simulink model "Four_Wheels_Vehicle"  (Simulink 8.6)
settings: Solver=ode45  StartTime=0.0  StopTime=20  RelTol=1e-3
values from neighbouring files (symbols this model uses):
  beta = 1    [Vehicle_Parameters.m]
  g = 9.81    [Vehicle_Parameters.m]
  H_CoG = 0.700    (= 0.7)    [Vehicle_Parameters.m]
  Hearo = 0.750    (= 0.75)    [Vehicle_Parameters.m]
  Iz = 2480    [Vehicle_Parameters.m]
  Jw = 2.166    [Vehicle_Parameters.m]
  L = 10    [Vehicle_Parameters.m]
  Lf = 1.180    (= 1.18)    [Vehicle_Parameters.m]
  Lr = 1.770    (= 1.77)    [Vehicle_Parameters.m]
  Lw = 1.880    (= 1.88)    [Vehicle_Parameters.m]
  m = 1500    [Vehicle_Parameters.m]
  miu = 0.85    [Vehicle_Parameters.m]
  reff = 0.380    (= 0.38)    [Vehicle_Parameters.m]
undefined symbols (not defined in the file or in its folder): DiscIntNeverNeededParam, Init, Ki, Kp, LowerLimit, sigbuilder_block, Ts, UpperLimit
libraries: simulink x15, powerlib_extras x3
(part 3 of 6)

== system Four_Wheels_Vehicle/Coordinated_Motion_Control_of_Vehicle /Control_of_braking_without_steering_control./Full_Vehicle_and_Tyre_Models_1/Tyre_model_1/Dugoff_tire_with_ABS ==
  note: Dugoff_Tire_model
  In1 : Inport
  In2 : Inport  Port=2
  In5 : Inport  Port=3
  In3 : Inport  Port=4
  Demux{1..4} (4 alike) : Demux  Outputs=3
  Dugoff_Tire_FL : MATLAB Function  TreatAsAtomicUnit=on
  Dugoff_Tire_FR : MATLAB Function  TreatAsAtomicUnit=on
  Dugoff_Tire_RL : MATLAB Function  TreatAsAtomicUnit=on
  Dugoff_Tire_RR : MATLAB Function  TreatAsAtomicUnit=on
  miu{,1..3} (4 alike) : Constant  Value=miu
  Fx_FL_1 : Outport
  Fx_FR_1 : Outport  Port=2
  Fy_FL_1 : Outport  Port=3
  Fy_FR_1 : Outport  Port=4
  Fx_RL_1 : Outport  Port=5
  Fx_RR_1 : Outport  Port=6
  Fy_RL_1 : Outport  Port=7
  Fy_RR_1 : Outport  Port=8
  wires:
  In3/1 -> Demux3/1
  Demux1/3 -> Dugoff_Tire_RR/3(alpha_RR)
  Demux1/1 -> Dugoff_Tire_RR/1(Sigma)
  Demux3/1 -> Dugoff_Tire_RL/1(Sigma)
  Demux3/3 -> Dugoff_Tire_RL/3(alpha_RL)
  In2/1 -> Demux2/1
  Dugoff_Tire_RR/2(Fy_RR) -> Fy_RR_1/1
  Dugoff_Tire_RL/2(Fy_RL) -> Fy_RL_1/1
  Dugoff_Tire_RR/1(Fx_RR) -> Fx_RR_1/1
  Dugoff_Tire_RL/1(Fx_RL) -> Fx_RL_1/1
  In5/1 -> Demux1/1
  Dugoff_Tire_FR/2(Fy_FR) -> Fy_FR_1/1
  Dugoff_Tire_FL/2(Fy_FL) -> Fy_FL_1/1
  Dugoff_Tire_FR/1(Fx_FR) -> Fx_FR_1/1
  Dugoff_Tire_FL/1(Fx_FL) -> Fx_FL_1/1
  In1/1 -> Demux4/1
  miu3/1 -> Dugoff_Tire_RR/4(miu)
  miu2/1 -> Dugoff_Tire_RL/4(miu)
  miu/1 -> Dugoff_Tire_FR/4(miu)
  miu1/1 -> Dugoff_Tire_FL/4(miu)
  Demux4/1 -> Dugoff_Tire_FL/1(Sigma)
  Demux4/2 -> Dugoff_Tire_FL/2(Fz_FL)
  Demux4/3 -> Dugoff_Tire_FL/3(alpha_FL)
  Demux3/2 -> Dugoff_Tire_RL/2(Fz_RL)
  Demux2/1 -> Dugoff_Tire_FR/1(Sigma)
  Demux2/2 -> Dugoff_Tire_FR/2(Fz_FR)
  Demux2/3 -> Dugoff_Tire_FR/3(alpha_FR)
  Demux1/2 -> Dugoff_Tire_RR/2(Fz_RR)

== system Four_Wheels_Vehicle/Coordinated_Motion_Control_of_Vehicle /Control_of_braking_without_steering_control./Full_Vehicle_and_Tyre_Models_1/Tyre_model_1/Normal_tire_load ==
  x_Vel_1 : Inport
  mass : Inport  Port=2
  g : Inport  Port=3
  H_CoG : Inport  Port=4
  beta : Inport  Port=5
  Lf : Inport  Port=6
  Lr : Inport  Port=7
  Hearo : Inport  Port=8
  AirDragConst : Constant  Value=0.3
  Airdensity : Constant  Value=1.22
  Constant : Constant  Value=2
  Constant1 : Constant  Value=2
  Divide : Product  Inputs=*/
  Divide1 : Product  Inputs=*/
  Faero : Subsystem
  FrontalArea : Constant  Value=2
  Fzf : Subsystem
  Fzr : Subsystem
  Scope : Scope
  windVelocity : Constant
  Fz_f_1 : Outport
  Fz_r_1 : Outport  Port=2
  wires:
  Faero/1(Faero) -> Scope/1, Fzf/9(Faero), Fzr/1(Faero)
  x_Vel_1/1 -> Fzr/3(xVel), Fzf/1(x_Vel), Faero/1(Vx)
  windVelocity/1 -> Faero/5(windVelocity)
  Airdensity/1 -> Faero/4(Airdensity)
  FrontalArea/1 -> Faero/3(FrontalArea1)
  AirDragConst/1 -> Faero/2(AirDragConst1)
  mass/1 -> Fzr/4(mass), Fzf/2(mass)
  Hearo/1 -> Fzr/2(Haero), Fzf/8(Haero)
  H_CoG/1 -> Fzr/6(HatCG), Fzf/4(H_CoG)
  g/1 -> Fzr/5(g), Fzf/3(g)
  Divide1/1 -> Fz_r_1/1
  Divide/1 -> Fz_f_1/1
  Constant1/1 -> Divide1/2
  Constant/1 -> Divide/2
  Fzr/1(Fzr) -> Divide1/1
  Fzf/1(Fz_f) -> Divide/1
  Lf/1 -> Fzr/8(Lf), Fzf/6(Lf)
  beta/1 -> Fzr/7(beta), Fzf/5(beta)
  Lr/1 -> Fzr/9(Lr), Fzf/7(Lr)

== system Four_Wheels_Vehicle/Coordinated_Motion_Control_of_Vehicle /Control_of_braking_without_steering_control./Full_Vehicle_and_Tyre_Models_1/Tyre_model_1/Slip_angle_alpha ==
  note: Slip_angle_alpha
  x_Vel_1 : Inport
  y_Vel_1 : Inport  Port=2
  yaw_rate_1 : Inport  Port=3
  Steering_Ang._1 : Inport  Port=4
  Lf : Constant  Value=Lf
  Lr : Constant  Value=Lr
  Slip_angle_alpha : MATLAB Function  TreatAsAtomicUnit=on
  alpha_FL_1 : Outport
  alpha_FR_1 : Outport  Port=2
  alpha_RL_1 : Outport  Port=3
  alpha_RR_1 : Outport  Port=4
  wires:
  Steering_Ang._1/1 -> Slip_angle_alpha/6(deltaw)
  Lr/1 -> Slip_angle_alpha/5(Lr)
  Lf/1 -> Slip_angle_alpha/4(Lf)
  yaw_rate_1/1 -> Slip_angle_alpha/3(yaw_rate)
  y_Vel_1/1 -> Slip_angle_alpha/2(y_Vel)
  x_Vel_1/1 -> Slip_angle_alpha/1(x_Vel)
  Slip_angle_alpha/1(alpha_FL) -> alpha_FL_1/1
  Slip_angle_alpha/2(alpha_FR) -> alpha_FR_1/1
  Slip_angle_alpha/3(alpha_RL) -> alpha_RL_1/1
  Slip_angle_alpha/4(alpha_RR) -> alpha_RR_1/1

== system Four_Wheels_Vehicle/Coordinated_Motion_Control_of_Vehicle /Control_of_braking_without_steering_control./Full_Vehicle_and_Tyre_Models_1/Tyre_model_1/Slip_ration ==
  note: Slip_ration
  Omega_FL_1 : Inport
  Omega_FR_1 : Inport  Port=2
  Omega_RL_1 : Inport  Port=3
  Omega_RR_1 : Inport  Port=4
  x_Vel_1 : Inport  Port=5
  Slip_ration_Sigma : MATLAB Function  TreatAsAtomicUnit=on
  reff : Constant  Value=reff
  Sigma_FL_1 : Outport
  Sigma_FR_1 : Outport  Port=2
  Sigma_RL_1 : Outport  Port=3
  Sigma_RR_1 : Outport  Port=4
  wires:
  x_Vel_1/1 -> Slip_ration_Sigma/5(x_Vel)
  Omega_FR_1/1 -> Slip_ration_Sigma/2(Omega_FR)
  Omega_RR_1/1 -> Slip_ration_Sigma/4(Omega_RR)
  Omega_RL_1/1 -> Slip_ration_Sigma/3(Omega_RL)
  Omega_FL_1/1 -> Slip_ration_Sigma/1(Omega_FL)
  Slip_ration_Sigma/1(Sigma_FL) -> Sigma_FL_1/1
  Slip_ration_Sigma/4(Sigma_RR) -> Sigma_RR_1/1
  Slip_ration_Sigma/3(Sigma_RL) -> Sigma_RL_1/1
  Slip_ration_Sigma/2(Sigma_FR) -> Sigma_FR_1/1
  reff/1 -> Slip_ration_Sigma/6(reff)

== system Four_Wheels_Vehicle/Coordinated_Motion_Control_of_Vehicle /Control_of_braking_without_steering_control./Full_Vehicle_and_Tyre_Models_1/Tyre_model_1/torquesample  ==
  Demux : Demux  Tag=STV Demux  Outputs=1
  FromWs : FromWorkspace  Tag=STV FromWs  VariableName=tuvar  SampleTime=0  SigBuilderData=DataTag4  VnvData=DataTag5
  Signal 1 : Outport  Tag=STV Outport
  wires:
  Demux/1 -> Signal 1/1
  FromWs/1 -> Demux/1

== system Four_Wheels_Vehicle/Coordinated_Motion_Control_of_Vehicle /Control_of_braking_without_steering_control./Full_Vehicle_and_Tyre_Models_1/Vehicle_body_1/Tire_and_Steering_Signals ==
  Steering_Ang. : Inport
  Fx_and_Fy : Inport  Port=2
  Demux : Demux  Outputs=8
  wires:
  Fx_and_Fy/1 -> Demux/1
  Demux/8 -> [Fy_RR_1]
  Demux/7 -> [Fy_RL_1]
  Demux/6 -> [Fx_RR_1]
  Demux/5 -> [Fx_RL_1]
  Demux/4 -> [Fy_FR_1]
  Demux/3 -> [Fy_FL_1]
  Demux/2 -> [Fx_FR_1]
  Demux/1 -> [Fx_FL_1]
  Steering_Ang./1 -> [SteeringAng_1]

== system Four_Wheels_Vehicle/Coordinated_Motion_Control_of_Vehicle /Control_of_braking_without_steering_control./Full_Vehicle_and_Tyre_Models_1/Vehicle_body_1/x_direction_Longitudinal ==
  note: x_direction_Longitudinal
  Fx_FL_1 : Inport
  Fx_FR_1 : Inport  Port=2
  Fy_FL_1 : Inport  Port=3
  Fy_FR_1 : Inport  Port=4
  Fx_RL_1 : Inport  Port=5
  Fx_RR_1 : Inport  Port=6
  Steering_Ang_1 : Inport  Port=7
  yaw_rate_1 : Inport  Port=8
  y_Vel_1 : Inport  Port=9
  1/m : Gain  Gain=1/1750
  Add : Sum
  Add1 : Sum
  Add2 : Sum  Inputs=+-++
  Add3 : Sum
  Product : Product
  Product1 : Product
  Product18 : Product
  Stop Simulation : Stop
  Vx0 : Integrator  InitialCondition=5  UpperSaturationLimit=100  LowerSaturationLimit=0  ShowSaturationPort=on
  cos_deltaw : Fcn  Expr=cos(u)
  sin_deltaw : Fcn  Expr=sin(u)
  x_Vel_1 : Outport
  x total force : Outport  Port=2
  dx : Outport  Port=3
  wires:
  Fx_RR_1/1 -> Add2/4
  Fx_RL_1/1 -> Add2/3
  Product1/1 -> Add2/2
  Product/1 -> Add2/1
  Fx_FR_1/1 -> Add/2
  Fx_FL_1/1 -> Add/1
  Fy_FR_1/1 -> Add1/2
  Fy_FL_1/1 -> Add1/1
  sin_deltaw/1 -> Product1/2
  Add1/1 -> Product1/1
  y_Vel_1/1 -> Product18/2
  yaw_rate_1/1 -> Product18/1
  Steering_Ang_1/1 -> sin_deltaw/1, cos_deltaw/1
  Add/1 -> Product/1
  cos_deltaw/1 -> Product/2
  Add2/1 -> x total force/1, 1/m/1
  1/m/1 -> Add3/1
  Add3/1 -> Vx0/1, dx/1
  Vx0/2 -> Stop Simulation/1
  Vx0/1 -> x_Vel_1/1
  Product18/1 -> Add3/2

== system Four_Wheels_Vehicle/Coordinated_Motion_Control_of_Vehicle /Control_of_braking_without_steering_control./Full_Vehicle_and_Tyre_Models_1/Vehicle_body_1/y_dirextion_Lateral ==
  note: y_dirextion_Lateral
  Fx_FL_1 : Inport
  Fx_FR_1 : Inport  Port=2
  Fy_FL_1 : Inport  Port=3
  Fy_FR_1 : Inport  Port=4
  Fy_RL_1 : Inport  Port=5
  Fy_RR_1 : Inport  Port=6
  Steering_Ang._1 : Inport  Port=7
  yaw_rate_1 : Inport  Port=8
  x_Vel_1 : Inport  Port=9
  1/m : Gain  Gain=1/1750
  Add1 : Sum
  Add12 : Sum
  Add15 : Sum  Inputs=++++
  Add2 : Sum  Inputs=+-
  Product1 : Product
  Product13 : Product
  Product3 : Product
  Vx0 : Integrator  UpperSaturationLimit=50/3.6  LowerSaturationLimit=eps
  cos_deltaw2 : Fcn  Expr=cos(u)
  sin_deltaw2 : Fcn  Expr=sin(u)
  y_Vel_1 : Outport
  y total force : Outport  Port=2
  dy : Outport  Port=3
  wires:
  Add2/1 -> Vx0/1, dy/1
  Fy_RL_1/1 -> Add15/3
  Fy_RR_1/1 -> Add15/4
  Product13/1 -> Add15/1
  Product1/1 -> Add15/2
  Fx_FR_1/1 -> Add12/2
  Fx_FL_1/1 -> Add12/1
  Fy_FR_1/1 -> Add1/2
  Fy_FL_1/1 -> Add1/1
  Product3/1 -> Add2/2
  x_Vel_1/1 -> Product3/2
  yaw_rate_1/1 -> Product3/1
  cos_deltaw2/1 -> Product1/2
  Add1/1 -> Product1/1
  Vx0/1 -> y_Vel_1/1
  1/m/1 -> Add2/1
  Add15/1 -> y total force/1, 1/m/1
  sin_deltaw2/1 -> Product13/2
  Add12/1 -> Product13/1
  Steering_Ang._1/1 -> cos_deltaw2/1, sin_deltaw2/1

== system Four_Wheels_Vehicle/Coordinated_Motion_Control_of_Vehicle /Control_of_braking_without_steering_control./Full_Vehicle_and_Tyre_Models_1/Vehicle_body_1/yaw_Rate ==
  note: yaw_Rate_and_z_torque
  Fx_FL_1 : Inport
  Fx_FR_1 : Inport  Port=2
  Fy_FL_1 : Inport  Port=3
  Fy_FR_1 : Inport  Port=4
  Fx_RL_1 : Inport  Port=5
  Fx_RR_1 : Inport  Port=6
  Fy_RL_1 : Inport  Port=7
  Fy_RR_1 : Inport  Port=8
  Steering_Ang._1 : Inport  Port=9
  1/Iz : Gain  Gain=1/Iz
  Add1 : Sum  Inputs=-+
  Add10 : Sum  Inputs=+++++-
  Add2 : Sum
  Add3 : Sum  Inputs=-+
  Add4 : Sum
  Add5 : Sum  Inputs=-+
  Add6 : Sum
  Integrator1 : Integrator  InitialCondition=eps  UpperSaturationLimit=50/3.6  LowerSaturationLimit=eps  ShowSaturationPort=on
  Lf : Constant  Value=Lf
  Lr : Constant  Value=Lr
  Lw/2 : Constant  Value=Lw/2
  Product{1..9,13} (10 alike) : Product
  Stop Simulation1 : Stop
  cosdeltaw1 : Fcn  Expr=cos(u)
  sindeltaw1 : Fcn  Expr=sin(u)
  yaw_rate_1 : Outport
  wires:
  Fy_RR_1/1 -> Add6/2
  Fy_RL_1/1 -> Add6/1
  Fx_RR_1/1 -> Add5/2
  Fx_RL_1/1 -> Add5/1
  Fx_FR_1/1 -> Add1/2, Add4/2
  Fx_FL_1/1 -> Add1/1, Add4/1
  Fy_FL_1/1 -> Add2/1, Add3/2
  Fy_FR_1/1 -> Add3/1, Add2/2
  Add10/1 -> 1/Iz/1
  Add3/1 -> Product6/2
  Product6/1 -> Product5/1
  Product5/1 -> Add10/4
  Product9/1 -> Add10/5
  Product8/1 -> Add10/6
  Product2/1 -> Add10/3
  Product7/1 -> Product13/2
  Product13/1 -> Add10/2
  Add6/1 -> Product8/1
  Add5/1 -> Product9/1
  Add2/1 -> Product7/1
  Product4/1 -> Product2/1
  Product1/1 -> Product3/1
  Integrator1/2 -> Stop Simulation1/1
  Integrator1/1 -> yaw_rate_1/1
  1/Iz/1 -> Integrator1/1
  Product3/1 -> Add10/1
  Lr/1 -> Product8/2
  Lw/2/1 -> Product9/2, Product2/2, Product5/2
  cosdeltaw1/1 -> Product4/2, Product7/2
  Add1/1 -> Product4/1
  Lf/1 -> Product13/1, Product3/2
  sindeltaw1/1 -> Product1/2, Product6/1
  Add4/1 -> Product1/1
  Steering_Ang._1/1 -> sindeltaw1/1, cosdeltaw1/1

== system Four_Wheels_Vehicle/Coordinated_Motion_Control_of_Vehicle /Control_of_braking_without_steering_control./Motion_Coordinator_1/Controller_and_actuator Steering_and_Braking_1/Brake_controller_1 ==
  Reference_Sideslip_1 : Inport
  Feedback_Sideslip_1 : Inport  Port=2
  Add1 : Sum
  Brake_Actuator_1 : Subsystem
  Brake_controller_1 : Subsystem
  Ramp : simulink/Sources/Ramp  slope=3  start=1  X0=0
  Sideslip_angle : Scope  NumInputPorts=2
  x_seitch2 : ManualSwitch  CurrentSetting=0
  Mzc_1 : Outport
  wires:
  x_seitch2/1 -> Add1/2
  Add1/1 -> Mzc_1/1
  Reference_Sideslip_1/1 -> Brake_controller_1/1(Reference), Sideslip_angle/1, Add1/1
  Brake_controller_1/2(Sideslip_Ang1) -> Brake_Actuator_1/1(input)
  Feedback_Sideslip_1/1 -> Brake_controller_1/2(Feedback), Sideslip_angle/2
  Ramp/1 -> x_seitch2/1
  Brake_Actuator_1/1(output) -> x_seitch2/2

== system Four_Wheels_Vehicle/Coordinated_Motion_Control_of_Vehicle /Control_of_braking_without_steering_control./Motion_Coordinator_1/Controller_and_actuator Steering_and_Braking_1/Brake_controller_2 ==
  Reference_Sideslip_2 : Inport
  Feedback_Sideslip_2 : Inport  Port=2
  Add1 : Sum
  Brake_Actuator_2 : Subsystem
  Brake_controller_2 : Subsystem
  Ramp : simulink/Sources/Ramp  slope=3  start=1  X0=0
  Sideslip_angle : Scope  NumInputPorts=2
  x_seitch2 : ManualSwitch  CurrentSetting=0
  Mzc_2 : Outport
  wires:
  Brake_Actuator_2/1(output) -> x_seitch2/2
  Ramp/1 -> x_seitch2/1
  Feedback_Sideslip_2/1 -> Sideslip_angle/2, Brake_controller_2/2(Feedback)
  Brake_controller_2/2(Sideslip_Ang1) -> Brake_Actuator_2/1(input)
  Reference_Sideslip_2/1 -> Add1/1, Sideslip_angle/1, Brake_controller_2/1(Reference)
  Add1/1 -> Mzc_2/1
  x_seitch2/1 -> Add1/2

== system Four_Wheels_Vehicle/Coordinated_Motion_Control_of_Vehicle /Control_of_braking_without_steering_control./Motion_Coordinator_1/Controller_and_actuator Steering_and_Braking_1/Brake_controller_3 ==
  Reference_Sideslip_3 : Inport
  Feedback_Sideslip_3 : Inport  Port=2
  Add1 : Sum
  Brake_Actuator_3 : Subsystem
  Brake_controller_3 : Subsystem
  Ramp : simulink/Sources/Ramp  slope=3  start=1  X0=0
  Sideslip_angle : Scope  NumInputPorts=2
  x_seitch2 : ManualSwitch  CurrentSetting=0
  Mzc_3 : Outport
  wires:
  x_seitch2/1 -> Add1/2
  Add1/1 -> Mzc_3/1
  Reference_Sideslip_3/1 -> Brake_controller_3/1(Reference), Sideslip_angle/1, Add1/1
  Brake_controller_3/2(Sideslip_Ang1) -> Brake_Actuator_3/1(input)
  Feedback_Sideslip_3/1 -> Brake_controller_3/2(Feedback), Sideslip_angle/2
  Ramp/1 -> x_seitch2/1
  Brake_Actuator_3/1(output) -> x_seitch2/2

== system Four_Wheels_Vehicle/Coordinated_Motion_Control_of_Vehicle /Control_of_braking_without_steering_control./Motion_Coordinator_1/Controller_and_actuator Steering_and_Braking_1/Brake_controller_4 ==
  Reference_Sideslip_4 : Inport
  Feedback_Sideslip_4 : Inport  Port=2
  Add1 : Sum
  Brake_Actuator_4 : Subsystem
  Brake_controller_4 : Subsystem
  Ramp : simulink/Sources/Ramp  slope=3  start=1  X0=0
  Sideslip_angle : Scope  NumInputPorts=2
  x_seitch2 : ManualSwitch  CurrentSetting=0
  Mzc_4 : Outport
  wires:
  Brake_Actuator_4/1(output) -> x_seitch2/2
  Ramp/1 -> x_seitch2/1
  Feedback_Sideslip_4/1 -> Sideslip_angle/2, Brake_controller_4/2(Feedback)
  Brake_controller_4/2(Sideslip_Ang1) -> Brake_Actuator_4/1(input)
  Reference_Sideslip_4/1 -> Add1/1, Sideslip_angle/1, Brake_controller_4/1(Reference)
  Add1/1 -> Mzc_4/1
  x_seitch2/1 -> Add1/2

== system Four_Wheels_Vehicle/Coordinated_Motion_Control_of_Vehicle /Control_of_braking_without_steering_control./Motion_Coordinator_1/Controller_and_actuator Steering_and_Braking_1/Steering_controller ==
  StteringAng : Inport
  Reference_Steering : Inport  Port=2
  Feedback_Steering : Inport  Port=3
  Add : Sum
  Steering_Actuator : Subsystem
  Steering_controller : Subsystem
  x_seitch1 : ManualSwitch
  yaw_comparsion : Scope  NumInputPorts=2
  f : Outport
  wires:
  Reference_Steering/1 -> yaw_comparsion/1, Steering_controller/1(Reference), x_seitch1/1
  StteringAng/1 -> Add/1
  x_seitch1/1 -> Add/2
  Steering_controller/2(Steering_Ang1) -> Steering_Actuator/1(input)
  Steering_Actuator/1(output) -> x_seitch1/2
  Feedback_Steering/1 -> Steering_controller/2(Feedback), yaw_comparsion/2
  Add/1 -> f/1

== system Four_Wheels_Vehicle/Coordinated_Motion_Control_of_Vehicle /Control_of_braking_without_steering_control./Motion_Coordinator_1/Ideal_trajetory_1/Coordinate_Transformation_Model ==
  note: vehicle heading
  delta_steer (rad) : Inport
  v_x (m/s) : Inport  Port=2
  1/L : Gain  Gain=1/L
  Beta : Scope
  Beta1 : Scope
  Divide : Product  Inputs=*/
  Gain : Gain  Gain=L/2
  Gain1 : Gain  Gain=0.1
  Gain2 : Gain  Gain=0.1
  Gain4 : Gain  Gain=0.345
  Ground : Ground
  Integrator : Integrator
  Integrator1 : Integrator  LimitOutput=on  UpperSaturationLimit=0
  Integrator2 : Integrator
  Product{,1,3..4} (4 alike) : Product
  Sideslip_angle : Scope
  Subtract : Sum  Inputs=+-
  Sum : Sum  Inputs=|+-
  Sum1 : Sum  Inputs=|++
  Terminator : Terminator
  Trigonometric Function : Trigonometry  Operator=cos
  Trigonometric Function1 : Trigonometry
  Trigonometric Function2 : Trigonometry  Operator=atan
  Trigonometric Function3 : Trigonometry  Operator=tan
  steerVsYawrate1 : Scope  NumInputPorts=3
  steerVsYawrate2 : Scope  NumInputPorts=3
  yaw_rate : Product
  X-position : Outport
  Y-position : Outport  Port=2
  yaw_Rate : Outport  Port=3
  Sideslip_beta : Outport  Port=4
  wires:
  Product/1 -> Sum1/1
  Product1/1 -> Sum/1
  Trigonometric Function/1 -> Product1/2, Product4/2  "cos(psi)"
  Trigonometric Function1/1 -> Product/2, Product3/2  "sin(psi)"
  Integrator2/1 -> Gain1/1  "yaw_heading (rad)"
  Integrator/1 -> steerVsYawrate1/1, X-position/1
  Integrator1/1 -> steerVsYawrate1/2, Y-position/1
  v_x (m/s)/1 -> Product/1, Product1/1, 1/L/1  "v_x (m/s)"
  yaw_rate/1 -> steerVsYawrate2/1, Gain/1, Beta1/1, Subtract/2, yaw_Rate/1, Gain2/1
  1/L/1 -> yaw_rate/1  "v_x / L"
  Sum/1 -> steerVsYawrate2/2, Integrator/1, Divide/2  "v_X (m/s)"
  Sum1/1 -> Gain4/1  "v_Y (m/s)"
  Gain/1 -> Product3/1, Product4/1  "L/2*psi-dot"
  Product3/1 -> Sum/2
  Product4/1 -> Sum1/2
  Ground/1 -> Trigonometric Function3/1
  Trigonometric Function3/1 -> Terminator/1
  Divide/1 -> Trigonometric Function2/1
  delta_steer (rad)/1 -> yaw_rate/2
  Gain1/1 -> Trigonometric Function/1, steerVsYawrate1/3, Trigonometric Function1/1
  Gain2/1 -> Integrator2/1
  Trigonometric Function2/1 -> Sideslip_angle/1, Sideslip_beta/1, Subtract/1
  Gain4/1 -> steerVsYawrate2/3, Integrator1/1, Divide/1
  Subtract/1 -> Beta/1

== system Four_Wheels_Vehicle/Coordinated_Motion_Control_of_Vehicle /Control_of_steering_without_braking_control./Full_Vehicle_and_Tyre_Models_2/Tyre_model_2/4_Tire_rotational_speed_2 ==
  Tb_FL_2 : Inport
  Tb_FR_2 : Inport  Port=2
  Tb_RL_2 : Inport  Port=3
  Tb_RR_2 : Inport  Port=4
  Td_FL_2 : Inport  Port=5
  Td_FR_2 : Inport  Port=6
  Td_RL_2 : Inport  Port=7
  Td_RR_2 : Inport  Port=8
  Fx_FL_2 : Inport  Port=9
  Fx_FR_2 : Inport  Port=10
  Fx_RL_2 : Inport  Port=11
  Fx_RR_2 : Inport  Port=12
  Tire_speed_FL : Subsystem
  Tire_speed_FR : Subsystem
  Tire_speed_RL : Subsystem
  Tire_speed_RR : Subsystem
  Omega_FL_2 : Outport
  Omega_FR_2 : Outport  Port=2
  Omega_RL_2 : Outport  Port=3
  Omega_RR_2 : Outport  Port=4
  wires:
  Tb_FL_2/1 -> Tire_speed_FL/1(Tb_FL_2)
  Td_FL_2/1 -> Tire_speed_FL/2(Td_FL_2)
  Fx_FL_2/1 -> Tire_speed_FL/3(Fx_FL_2)
  Tire_speed_FL/1(Omega_FL_2) -> Omega_FL_2/1
  Tb_FR_2/1 -> Tire_speed_FR/1(Tb_FR_2)
  Td_FR_2/1 -> Tire_speed_FR/2(Td_FR_2)
  Fx_FR_2/1 -> Tire_speed_FR/3(Fx_FR_2)
  Tire_speed_FR/1(Omega_FR_2) -> Omega_FR_2/1
  Tb_RL_2/1 -> Tire_speed_RL/1(Tb_RL_2)
  Fx_RL_2/1 -> Tire_speed_RL/3(Fx_RL_2)
  Tire_speed_RL/1(Omega_RL_2) -> Omega_RL_2/1
  Tb_RR_2/1 -> Tire_speed_RR/1(Tb_RR_2)
  Fx_RR_2/1 -> Tire_speed_RR/3(Fx_RR_2)
  Tire_speed_RR/1(Omega_RR_2) -> Omega_RR_2/1
  Td_RL_2/1 -> Tire_speed_RL/2(Td_RL_2)
  Td_RR_2/1 -> Tire_speed_RR/2(Td_RR_2)

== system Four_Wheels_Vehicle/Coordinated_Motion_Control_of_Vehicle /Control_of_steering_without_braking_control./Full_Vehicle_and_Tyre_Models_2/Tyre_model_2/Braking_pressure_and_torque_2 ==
  Mzc_all_2 : Inport
  SteeringAng : Inport  Port=2
  Braking_pressure_and_torque_FL : MATLAB Function  TreatAsAtomicUnit=on
  Braking_pressure_and_torque_FR : MATLAB Function  TreatAsAtomicUnit=on
  Braking_pressure_and_torque_RL : MATLAB Function  TreatAsAtomicUnit=on
  Braking_pressure_and_torque_RR : MATLAB Function  TreatAsAtomicUnit=on
  Demux : Demux
  reff{,1..3} (4 alike) : Constant  Value=reff
  tw{,1..3} (4 alike) : Constant  Value=1.65
  Tb_FL_2 : Outport
  Tb_FR_2 : Outport  Port=2
  Tb_RL_2 : Outport  Port=3
  Tb_RR_2 : Outport  Port=4
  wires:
  Braking_pressure_and_torque_FR/2(Tb_FR) -> Tb_FR_2/1
  reff1/1 -> Braking_pressure_and_torque_FR/2(reff)
  reff3/1 -> Braking_pressure_and_torque_RR/2(reff)
  tw2/1 -> Braking_pressure_and_torque_RL/3(tw)
  Braking_pressure_and_torque_RR/2(Tb_RR) -> Tb_RR_2/1
  reff/1 -> Braking_pressure_and_torque_FL/2(reff)
  Braking_pressure_and_torque_FL/2(Tb_FL) -> Tb_FL_2/1
  tw3/1 -> Braking_pressure_and_torque_RR/3(tw)
  tw1/1 -> Braking_pressure_and_torque_FR/3(tw)
  reff2/1 -> Braking_pressure_and_torque_RL/2(reff)
  Braking_pressure_and_torque_RL/2(Tb_RL) -> Tb_RL_2/1
  tw/1 -> Braking_pressure_and_torque_FL/3(tw)
  SteeringAng/1 -> Braking_pressure_and_torque_FR/4(SteeringAng), Braking_pressure_and_torque_FL/4(SteeringAng)
  Mzc_all_2/1 -> Demux/1
  Demux/1 -> Braking_pressure_and_torque_FL/1(M)
  Demux/2 -> Braking_pressure_and_torque_FR/1(M)
  Demux/3 -> Braking_pressure_and_torque_RL/1(M)
  Demux/4 -> Braking_pressure_and_torque_RR/1(M)

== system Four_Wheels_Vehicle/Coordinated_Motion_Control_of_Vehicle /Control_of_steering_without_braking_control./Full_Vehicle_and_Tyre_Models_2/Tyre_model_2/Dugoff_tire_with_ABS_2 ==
  note: Dugoff_Tire_model
  In1 : Inport
  In2 : Inport  Port=2
  In5 : Inport  Port=3
  In3 : Inport  Port=4
  Demux{1..4} (4 alike) : Demux  Outputs=3
  Dugoff_Tire_FL : MATLAB Function  TreatAsAtomicUnit=on
  Dugoff_Tire_FR : MATLAB Function  TreatAsAtomicUnit=on
  Dugoff_Tire_RL : MATLAB Function  TreatAsAtomicUnit=on
  Dugoff_Tire_RR : MATLAB Function  TreatAsAtomicUnit=on
  miu{,1..3} (4 alike) : Constant  Value=miu
  Fx_FL_2 : Outport
  Fx_FR_2 : Outport  Port=2
  Fy_FL_2 : Outport  Port=3
  Fy_FR_2 : Outport  Port=4
  Fx_RL_2 : Outport  Port=5
  Fx_RR_2 : Outport  Port=6
  Fy_RL_2 : Outport  Port=7
  Fy_RR_2 : Outport  Port=8
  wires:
  Demux1/2 -> Dugoff_Tire_RR/2(Fz_RR)
  Demux2/3 -> Dugoff_Tire_FR/3(alpha_FR)
  Demux2/2 -> Dugoff_Tire_FR/2(Fz_FR)
  Demux2/1 -> Dugoff_Tire_FR/1(Sigma)
  Demux3/2 -> Dugoff_Tire_RL/2(Fz_RL)
  Demux4/3 -> Dugoff_Tire_FL/3(alpha_FL)
  Demux4/2 -> Dugoff_Tire_FL/2(Fz_FL)
  Demux4/1 -> Dugoff_Tire_FL/1(Sigma)
  miu1/1 -> Dugoff_Tire_FL/4(miu)
  miu/1 -> Dugoff_Tire_FR/4(miu)
  miu2/1 -> Dugoff_Tire_RL/4(miu)
  miu3/1 -> Dugoff_Tire_RR/4(miu)
  In1/1 -> Demux4/1
  Dugoff_Tire_FL/1(Fx_FL) -> Fx_FL_2/1
  Dugoff_Tire_FR/1(Fx_FR) -> Fx_FR_2/1
  Dugoff_Tire_FL/2(Fy_FL) -> Fy_FL_2/1
  Dugoff_Tire_FR/2(Fy_FR) -> Fy_FR_2/1
  In5/1 -> Demux1/1
  Dugoff_Tire_RL/1(Fx_RL) -> Fx_RL_2/1
  Dugoff_Tire_RR/1(Fx_RR) -> Fx_RR_2/1
  Dugoff_Tire_RL/2(Fy_RL) -> Fy_RL_2/1
  Dugoff_Tire_RR/2(Fy_RR) -> Fy_RR_2/1
  In2/1 -> Demux2/1
  Demux3/3 -> Dugoff_Tire_RL/3(alpha_RL)
  Demux3/1 -> Dugoff_Tire_RL/1(Sigma)
  Demux1/1 -> Dugoff_Tire_RR/1(Sigma)
  Demux1/3 -> Dugoff_Tire_RR/3(alpha_RR)
  In3/1 -> Demux3/1

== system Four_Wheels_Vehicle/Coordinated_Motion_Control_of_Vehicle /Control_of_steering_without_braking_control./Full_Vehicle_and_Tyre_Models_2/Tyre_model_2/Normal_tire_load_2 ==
  x_Vel_2 : Inport
  mass : Inport  Port=2
  g : Inport  Port=3
  H_CoG : Inport  Port=4
  beta : Inport  Port=5
  Lf : Inport  Port=6
  Lr : Inport  Port=7
  Hearo : Inport  Port=8
  AirDragConst : Constant  Value=0.3
  Airdensity : Constant  Value=1.22
  Constant : Constant  Value=2
  Constant1 : Constant  Value=2
  Divide : Product  Inputs=*/
  Divide1 : Product  Inputs=*/
  Faero : Subsystem
  FrontalArea : Constant  Value=2
  Fzf_2 : Subsystem
  Fzr_2 : Subsystem
  Scope : Scope
  windVelocity : Constant
  Fz_f_2 : Outport
  Fz_r_2 : Outport  Port=2
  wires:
  Lr/1 -> Fzf_2/7(Lr), Fzr_2/9(Lr)
  beta/1 -> Fzf_2/5(beta), Fzr_2/7(beta)
  Lf/1 -> Fzf_2/6(Lf), Fzr_2/8(Lf)
  Fzf_2/1(Fz_f) -> Divide/1
  Fzr_2/1(Fzr) -> Divide1/1
  Constant/1 -> Divide/2
  Constant1/1 -> Divide1/2
  Divide/1 -> Fz_f_2/1
  Divide1/1 -> Fz_r_2/1
  g/1 -> Fzf_2/3(g), Fzr_2/5(g)
  H_CoG/1 -> Fzf_2/4(H_CoG), Fzr_2/6(HatCG)
  Hearo/1 -> Fzf_2/8(Haero), Fzr_2/2(Haero)
  mass/1 -> Fzf_2/2(mass), Fzr_2/4(mass)
  AirDragConst/1 -> Faero/2(AirDragConst1)
  FrontalArea/1 -> Faero/3(FrontalArea1)
  Airdensity/1 -> Faero/4(Airdensity)
  windVelocity/1 -> Faero/5(windVelocity)
  x_Vel_2/1 -> Faero/1(Vx), Fzf_2/1(x_Vel), Fzr_2/3(xVel)
  Faero/1(Faero) -> Fzr_2/1(Faero), Fzf_2/9(Faero), Scope/1

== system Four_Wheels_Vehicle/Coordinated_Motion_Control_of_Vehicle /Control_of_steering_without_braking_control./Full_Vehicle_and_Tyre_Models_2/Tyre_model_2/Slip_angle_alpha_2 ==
  note: Slip_angle_alpha
  x_Vel_2 : Inport
  y_Vel_2 : Inport  Port=2
  yaw_rate_2 : Inport  Port=3
  Steering_Ang._2 : Inport  Port=4
  Lf : Constant  Value=Lf
  Lr : Constant  Value=Lr
  Slip_angle_alpha : MATLAB Function  TreatAsAtomicUnit=on
  alpha_FL_2 : Outport
  alpha_FR_2 : Outport  Port=2
  alpha_RL_2 : Outport  Port=3
  alpha_RR_2 : Outport  Port=4
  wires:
  Slip_angle_alpha/4(alpha_RR) -> alpha_RR_2/1
  Slip_angle_alpha/3(alpha_RL) -> alpha_RL_2/1
  Slip_angle_alpha/2(alpha_FR) -> alpha_FR_2/1
  Slip_angle_alpha/1(alpha_FL) -> alpha_FL_2/1
  x_Vel_2/1 -> Slip_angle_alpha/1(x_Vel)
  y_Vel_2/1 -> Slip_angle_alpha/2(y_Vel)
  yaw_rate_2/1 -> Slip_angle_alpha/3(yaw_rate)
  Lf/1 -> Slip_angle_alpha/4(Lf)
  Lr/1 -> Slip_angle_alpha/5(Lr)
  Steering_Ang._2/1 -> Slip_angle_alpha/6(deltaw)

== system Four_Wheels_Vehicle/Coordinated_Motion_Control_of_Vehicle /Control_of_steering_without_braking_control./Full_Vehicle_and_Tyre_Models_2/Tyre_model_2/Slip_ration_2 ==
  note: Slip_ration
  Omega_FL_2 : Inport
  Omega_FR_2 : Inport  Port=2
  Omega_RL_2 : Inport  Port=3
  Omega_RR_2 : Inport  Port=4
  x_Vel_2 : Inport  Port=5
  Slip_ration_Sigma_2 : MATLAB Function  TreatAsAtomicUnit=on
  reff : Constant  Value=reff
  Sigma_FL_2 : Outport
  Sigma_FR_2 : Outport  Port=2
  Sigma_RL_2 : Outport  Port=3
  Sigma_RR_2 : Outport  Port=4
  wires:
  reff/1 -> Slip_ration_Sigma_2/6(reff)
  Slip_ration_Sigma_2/2(Sigma_FR) -> Sigma_FR_2/1
  Slip_ration_Sigma_2/3(Sigma_RL) -> Sigma_RL_2/1
  Slip_ration_Sigma_2/4(Sigma_RR) -> Sigma_RR_2/1
  Slip_ration_Sigma_2/1(Sigma_FL) -> Sigma_FL_2/1
  Omega_FL_2/1 -> Slip_ration_Sigma_2/1(Omega_FL)
  Omega_RL_2/1 -> Slip_ration_Sigma_2/3(Omega_RL)
  Omega_RR_2/1 -> Slip_ration_Sigma_2/4(Omega_RR)
  Omega_FR_2/1 -> Slip_ration_Sigma_2/2(Omega_FR)
  x_Vel_2/1 -> Slip_ration_Sigma_2/5(x_Vel)

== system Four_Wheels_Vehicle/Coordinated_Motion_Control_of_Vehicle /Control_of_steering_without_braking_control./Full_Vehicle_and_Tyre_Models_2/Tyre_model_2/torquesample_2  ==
  Demux : Demux  Tag=STV Demux  Outputs=1
  FromWs : FromWorkspace  Tag=STV FromWs  VariableName=tuvar  SampleTime=0  SigBuilderData=DataTag10  VnvData=DataTag11
  Signal 1 : Outport  Tag=STV Outport
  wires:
  FromWs/1 -> Demux/1
  Demux/1 -> Signal 1/1

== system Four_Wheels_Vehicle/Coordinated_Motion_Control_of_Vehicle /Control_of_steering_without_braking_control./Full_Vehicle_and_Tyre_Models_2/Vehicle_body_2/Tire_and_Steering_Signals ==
  Steering_Ang._2 : Inport
  Fx_and_Fy_2 : Inport  Port=2
  Demux : Demux  Outputs=8
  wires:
  Steering_Ang._2/1 -> [SteeringAng_2]
  Demux/1 -> [Fx_FL_2]
  Demux/2 -> [Fx_FR_2]
  Demux/3 -> [Fy_FL_2]
  Demux/4 -> [Fy_FR_2]
  Demux/5 -> [Fx_RL_2]
  Demux/6 -> [Fx_RR_2]
  Demux/7 -> [Fy_RL_2]
  Demux/8 -> [Fy_RR_2]
  Fx_and_Fy_2/1 -> Demux/1

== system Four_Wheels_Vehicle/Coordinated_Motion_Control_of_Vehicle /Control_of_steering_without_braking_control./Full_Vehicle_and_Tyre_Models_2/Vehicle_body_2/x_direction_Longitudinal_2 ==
  note: x_direction_Longitudinal
  Fx_FL_2 : Inport
  Fx_FR_2 : Inport  Port=2
  Fy_FL_2 : Inport  Port=3
  Fy_FR_2 : Inport  Port=4
  Fx_RL_2 : Inport  Port=5
  Fx_RR_2 : Inport  Port=6
  Steering_Ang._2 : Inport  Port=7
  yaw_rate_2 : Inport  Port=8
  y_Vel_2 : Inport  Port=9
  1/m : Gain  Gain=1/1750
  Add : Sum
  Add1 : Sum
  Add2 : Sum  Inputs=+-++
  Add3 : Sum
  Product : Product
  Product1 : Product
  Product18 : Product
  Stop Simulation : Stop
  Vx0 : Integrator  InitialCondition=5  UpperSaturationLimit=100  LowerSaturationLimit=0  ShowSaturationPort=on
  cos_deltaw : Fcn  Expr=cos(u)
  sin_deltaw : Fcn  Expr=sin(u)
  x_Vel_2 : Outport
  x total force : Outport  Port=2
  dx : Outport  Port=3
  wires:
  Product18/1 -> Add3/2
  Vx0/1 -> x_Vel_2/1
  Vx0/2 -> Stop Simulation/1
  Add3/1 -> dx/1, Vx0/1
  1/m/1 -> Add3/1
  Add2/1 -> 1/m/1, x total force/1
  cos_deltaw/1 -> Product/2
  Add/1 -> Product/1
  Steering_Ang._2/1 -> cos_deltaw/1, sin_deltaw/1
  yaw_rate_2/1 -> Product18/1
  y_Vel_2/1 -> Product18/2
  Add1/1 -> Product1/1
  sin_deltaw/1 -> Product1/2
  Fy_FL_2/1 -> Add1/1
  Fy_FR_2/1 -> Add1/2
  Fx_FL_2/1 -> Add/1
  Fx_FR_2/1 -> Add/2
  Product/1 -> Add2/1
  Product1/1 -> Add2/2
  Fx_RL_2/1 -> Add2/3
  Fx_RR_2/1 -> Add2/4

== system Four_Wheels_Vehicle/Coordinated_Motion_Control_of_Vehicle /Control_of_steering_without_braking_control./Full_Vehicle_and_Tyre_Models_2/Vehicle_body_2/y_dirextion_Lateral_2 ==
  note: y_dirextion_Lateral
  Fx_FL_2 : Inport
  Fx_FR_2 : Inport  Port=2
  Fy_FL_2 : Inport  Port=3
  Fy_FR_2 : Inport  Port=4
  Fy_RL_2 : Inport  Port=5
  Fy_RR_2 : Inport  Port=6
  Steering_Ang._2 : Inport  Port=7
  yaw_rate_2 : Inport  Port=8
  x_Vel_2 : Inport  Port=9
  1/m : Gain  Gain=1/1750
  Add1 : Sum
  Add12 : Sum
  Add15 : Sum  Inputs=++++
  Add2 : Sum  Inputs=+-
  Product1 : Product
  Product13 : Product
  Product3 : Product
  Vx0 : Integrator  UpperSaturationLimit=50/3.6  LowerSaturationLimit=eps
  cos_deltaw2 : Fcn  Expr=cos(u)
  sin_deltaw2 : Fcn  Expr=sin(u)
  y_Vel_2 : Outport
  y total force : Outport  Port=2
  dy : Outport  Port=3
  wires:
  Steering_Ang._2/1 -> sin_deltaw2/1, cos_deltaw2/1
  Add12/1 -> Product13/1
  sin_deltaw2/1 -> Product13/2
  Add15/1 -> 1/m/1, y total force/1
  1/m/1 -> Add2/1
  Vx0/1 -> y_Vel_2/1
  Add1/1 -> Product1/1
  cos_deltaw2/1 -> Product1/2
  yaw_rate_2/1 -> Product3/1
  x_Vel_2/1 -> Product3/2
  Product3/1 -> Add2/2
  Fy_FL_2/1 -> Add1/1
  Fy_FR_2/1 -> Add1/2
  Fx_FL_2/1 -> Add12/1
  Fx_FR_2/1 -> Add12/2
  Product1/1 -> Add15/2
  Product13/1 -> Add15/1
  Fy_RR_2/1 -> Add15/4
  Fy_RL_2/1 -> Add15/3
  Add2/1 -> dy/1, Vx0/1

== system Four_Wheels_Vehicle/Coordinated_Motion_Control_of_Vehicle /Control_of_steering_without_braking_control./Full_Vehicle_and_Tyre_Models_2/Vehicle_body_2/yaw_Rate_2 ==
  note: yaw_Rate_and_z_torque
  Fx_FL_2 : Inport
  Fx_FR_2 : Inport  Port=2
  Fy_FL_2 : Inport  Port=3
  Fy_FR_2 : Inport  Port=4
  Fx_RL_2 : Inport  Port=5
  Fx_RR_2 : Inport  Port=6
  Fy_RL_2 : Inport  Port=7
  Fy_RR_2 : Inport  Port=8
  Steering_Ang._2 : Inport  Port=9
  1/Iz : Gain  Gain=1/Iz
  Add1 : Sum  Inputs=-+
  Add10 : Sum  Inputs=+++++-
  Add2 : Sum
  Add3 : Sum  Inputs=-+
  Add4 : Sum
  Add5 : Sum  Inputs=-+
  Add6 : Sum
  Integrator1 : Integrator  InitialCondition=eps  UpperSaturationLimit=50/3.6  LowerSaturationLimit=eps  ShowSaturationPort=on
  Lf : Constant  Value=Lf
  Lr : Constant  Value=Lr
  Lw/2 : Constant  Value=Lw/2
  Product{1..9,13} (10 alike) : Product
  Stop Simulation1 : Stop
  cosdeltaw1 : Fcn  Expr=cos(u)
  sindeltaw1 : Fcn  Expr=sin(u)
  yaw_rate_2 : Outport
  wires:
  Steering_Ang._2/1 -> cosdeltaw1/1, sindeltaw1/1
  Add4/1 -> Product1/1
  sindeltaw1/1 -> Product6/1, Product1/2
  Lf/1 -> Product3/2, Product13/1
  Add1/1 -> Product4/1
  cosdeltaw1/1 -> Product7/2, Product4/2
  Lw/2/1 -> Product5/2, Product2/2, Product9/2
  Lr/1 -> Product8/2
  Product3/1 -> Add10/1
  1/Iz/1 -> Integrator1/1
  Integrator1/1 -> yaw_rate_2/1
  Integrator1/2 -> Stop Simulation1/1
  Product1/1 -> Product3/1
  Product4/1 -> Product2/1
  Add2/1 -> Product7/1
  Add5/1 -> Product9/1
  Add6/1 -> Product8/1
  Product13/1 -> Add10/2
  Product7/1 -> Product13/2
  Product2/1 -> Add10/3
  Product8/1 -> Add10/6
  Product9/1 -> Add10/5
  Product5/1 -> Add10/4
  Product6/1 -> Product5/1
  Add3/1 -> Product6/2
  Add10/1 -> 1/Iz/1
  Fy_FR_2/1 -> Add2/2, Add3/1
  Fy_FL_2/1 -> Add3/2, Add2/1
  Fx_FL_2/1 -> Add4/1, Add1/1
  Fx_FR_2/1 -> Add4/2, Add1/2
  Fx_RL_2/1 -> Add5/1
  Fx_RR_2/1 -> Add5/2
  Fy_RL_2/1 -> Add6/1
  Fy_RR_2/1 -> Add6/2

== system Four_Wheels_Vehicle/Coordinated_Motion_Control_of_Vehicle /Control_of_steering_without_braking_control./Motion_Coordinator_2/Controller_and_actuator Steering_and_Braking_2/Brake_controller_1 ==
  Reference_Sideslip_1 : Inport
  Feedback_Sideslip_1 : Inport  Port=2
  Add1 : Sum
  Brake_Actuator_1 : Subsystem
  Brake_controller_1 : Subsystem
  Ramp : simulink/Sources/Ramp  slope=4  start=1  X0=0
  Sideslip_angle : Scope  NumInputPorts=2
  x_seitch2 : ManualSwitch
  Mzc_1 : Outport
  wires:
  Brake_Actuator_1/1(output) -> x_seitch2/2
  Ramp/1 -> x_seitch2/1
  Feedback_Sideslip_1/1 -> Sideslip_angle/2, Brake_controller_1/2(Feedback)
  Brake_controller_1/2(Sideslip_Ang1) -> Brake_Actuator_1/1(input)
  Reference_Sideslip_1/1 -> Add1/1, Sideslip_angle/1, Brake_controller_1/1(Reference)
  Add1/1 -> Mzc_1/1
  x_seitch2/1 -> Add1/2

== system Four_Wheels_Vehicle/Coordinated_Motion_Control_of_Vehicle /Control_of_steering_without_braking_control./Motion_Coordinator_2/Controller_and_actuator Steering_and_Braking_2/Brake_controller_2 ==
  Reference_Sideslip_2 : Inport
  Feedback_Sideslip_2 : Inport  Port=2
  Add1 : Sum
  Brake_Actuator_2 : Subsystem
  Brake_controller_2 : Subsystem
  Ramp : simulink/Sources/Ramp  slope=3  start=1  X0=0
  Sideslip_angle : Scope  NumInputPorts=2
  x_seitch2 : ManualSwitch
  Mzc_2 : Outport
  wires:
  x_seitch2/1 -> Add1/2
  Add1/1 -> Mzc_2/1
  Reference_Sideslip_2/1 -> Brake_controller_2/1(Reference), Sideslip_angle/1, Add1/1
  Brake_controller_2/2(Sideslip_Ang1) -> Brake_Actuator_2/1(input)
  Feedback_Sideslip_2/1 -> Brake_controller_2/2(Feedback), Sideslip_angle/2
  Ramp/1 -> x_seitch2/1
  Brake_Actuator_2/1(output) -> x_seitch2/2

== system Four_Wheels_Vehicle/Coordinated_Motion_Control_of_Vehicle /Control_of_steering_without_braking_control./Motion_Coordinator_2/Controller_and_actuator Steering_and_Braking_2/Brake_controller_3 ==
  Reference_Sideslip_3 : Inport
  Feedback_Sideslip_3 : Inport  Port=2
  Add1 : Sum
  Brake_Actuator_3 : Subsystem
  Brake_controller_3 : Subsystem
  Ramp : simulink/Sources/Ramp  slope=3  start=1  X0=0
  Sideslip_angle : Scope  NumInputPorts=2
  x_seitch2 : ManualSwitch
  Mzc_3 : Outport
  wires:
  Brake_Actuator_3/1(output) -> x_seitch2/2
  Ramp/1 -> x_seitch2/1
  Feedback_Sideslip_3/1 -> Sideslip_angle/2, Brake_controller_3/2(Feedback)
  Brake_controller_3/2(Sideslip_Ang1) -> Brake_Actuator_3/1(input)
  Reference_Sideslip_3/1 -> Add1/1, Sideslip_angle/1, Brake_controller_3/1(Reference)
  Add1/1 -> Mzc_3/1
  x_seitch2/1 -> Add1/2

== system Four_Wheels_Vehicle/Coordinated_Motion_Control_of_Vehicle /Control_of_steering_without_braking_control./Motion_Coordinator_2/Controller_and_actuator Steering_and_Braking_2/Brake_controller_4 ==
  Reference_Sideslip_4 : Inport
  Feedback_Sideslip_4 : Inport  Port=2
  Add1 : Sum
  Brake_Actuator_4 : Subsystem
  Brake_controller_4 : Subsystem
  Ramp : simulink/Sources/Ramp  slope=3  start=1  X0=0
  Sideslip_angle : Scope  NumInputPorts=2
  x_seitch2 : ManualSwitch
  Mzc_4 : Outport
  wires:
  x_seitch2/1 -> Add1/2
  Add1/1 -> Mzc_4/1
  Reference_Sideslip_4/1 -> Brake_controller_4/1(Reference), Sideslip_angle/1, Add1/1
  Brake_controller_4/2(Sideslip_Ang1) -> Brake_Actuator_4/1(input)
  Feedback_Sideslip_4/1 -> Brake_controller_4/2(Feedback), Sideslip_angle/2
  Ramp/1 -> x_seitch2/1
  Brake_Actuator_4/1(output) -> x_seitch2/2

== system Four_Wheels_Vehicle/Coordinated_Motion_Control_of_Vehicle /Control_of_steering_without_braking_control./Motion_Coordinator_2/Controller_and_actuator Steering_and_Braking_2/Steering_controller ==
  StteringAng : Inport
  Reference_Steering : Inport  Port=2
  Feedback_Steering : Inport  Port=3
  Add : Sum
  Steering_Actuator : Subsystem
  Steering_controller : Subsystem
  x_seitch1 : ManualSwitch  CurrentSetting=0
  yaw_comparsion : Scope  NumInputPorts=2
  f : Outport
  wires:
  Add/1 -> f/1
  Feedback_Steering/1 -> yaw_comparsion/2, Steering_controller/2(Feedback)
  Steering_Actuator/1(output) -> x_seitch1/2
  Steering_controller/2(Steering_Ang1) -> Steering_Actuator/1(input)
  x_seitch1/1 -> Add/2
  StteringAng/1 -> Add/1
  Reference_Steering/1 -> x_seitch1/1, Steering_controller/1(Reference), yaw_comparsion/1

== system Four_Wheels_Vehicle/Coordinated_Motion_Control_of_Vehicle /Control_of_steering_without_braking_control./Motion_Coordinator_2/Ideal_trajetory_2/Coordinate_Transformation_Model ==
  note: vehicle heading
  delta_steer (rad) : Inport
  v_x (m/s) : Inport  Port=2
  1/L : Gain  Gain=1/L
  Beta : Scope
  Beta1 : Scope
  Divide : Product  Inputs=*/
  Gain : Gain  Gain=L/2
  Gain1 : Gain  Gain=0.1
  Gain2 : Gain  Gain=0.1
  Gain4 : Gain  Gain=0.345
  Ground : Ground
  Integrator : Integrator
  Integrator1 : Integrator  LimitOutput=on  UpperSaturationLimit=0
  Integrator2 : Integrator
  Product{,1,3..4} (4 alike) : Product
  Sideslip_angle : Scope
  Subtract : Sum  Inputs=+-
  Sum : Sum  Inputs=|+-
  Sum1 : Sum  Inputs=|++
  Terminator : Terminator
  Trigonometric Function : Trigonometry  Operator=cos
  Trigonometric Function1 : Trigonometry
  Trigonometric Function2 : Trigonometry  Operator=atan
  Trigonometric Function3 : Trigonometry  Operator=tan
  steerVsYawrate1 : Scope  NumInputPorts=3
  steerVsYawrate2 : Scope  NumInputPorts=3
  yaw_rate : Product
  X-position : Outport
  Y-position : Outport  Port=2
  yaw_Rate : Outport  Port=3
  Sideslip_beta : Outport  Port=4
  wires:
  Subtract/1 -> Beta/1
  Gain4/1 -> Divide/1, Integrator1/1, steerVsYawrate2/3
  Trigonometric Function2/1 -> Subtract/1, Sideslip_beta/1, Sideslip_angle/1
  Gain2/1 -> Integrator2/1
  Gain1/1 -> Trigonometric Function1/1, steerVsYawrate1/3, Trigonometric Function/1
  delta_steer (rad)/1 -> yaw_rate/2
  Divide/1 -> Trigonometric Function2/1
  Trigonometric Function3/1 -> Terminator/1
  Ground/1 -> Trigonometric Function3/1
  Product4/1 -> Sum1/2
  Product3/1 -> Sum/2
  Gain/1 -> Product4/1, Product3/1  "L/2*psi-dot"
  Sum1/1 -> Gain4/1  "v_Y (m/s)"
  Sum/1 -> Divide/2, Integrator/1, steerVsYawrate2/2  "v_X (m/s)"
  1/L/1 -> yaw_rate/1  "v_x / L"
  yaw_rate/1 -> Gain2/1, yaw_Rate/1, Subtract/2, Beta1/1, Gain/1, steerVsYawrate2/1
  v_x (m/s)/1 -> 1/L/1, Product1/1, Product/1  "v_x (m/s)"
  Integrator1/1 -> Y-position/1, steerVsYawrate1/2
  Integrator/1 -> X-position/1, steerVsYawrate1/1
  Integrator2/1 -> Gain1/1  "yaw_heading (rad)"
  Trigonometric Function1/1 -> Product3/2, Product/2  "sin(psi)"
  Trigonometric Function/1 -> Product4/2, Product1/2  "cos(psi)"
  Product1/1 -> Sum/1
  Product/1 -> Sum1/1

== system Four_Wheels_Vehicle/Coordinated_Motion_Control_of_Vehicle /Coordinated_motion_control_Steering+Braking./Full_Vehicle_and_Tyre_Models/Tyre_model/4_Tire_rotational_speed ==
  Tb_FL : Inport
  Tb_FR : Inport  Port=2
  Tb_RL : Inport  Port=3
  Tb_RR : Inport  Port=4
  Td_FL : Inport  Port=5
  Td_FR : Inport  Port=6
  Td_RL : Inport  Port=7
  Td_RR : Inport  Port=8
  Fx_FL : Inport  Port=9
  Fx_FR : Inport  Port=10
  Fx_RL : Inport  Port=11
  Fx_RR : Inport  Port=12
  Tire_speed_FL : Subsystem
  Tire_speed_FR : Subsystem
  Tire_speed_RL : Subsystem
  Tire_speed_RR : Subsystem
  Omega_FL : Outport
  Omega_FR : Outport  Port=2
  Omega_RL : Outport  Port=3
  Omega_RR : Outport  Port=4
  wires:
  Tb_FL/1 -> Tire_speed_FL/1(Tb_FL)
  Td_FL/1 -> Tire_speed_FL/2(Td_FL)
  Fx_FL/1 -> Tire_speed_FL/3(Fx_FL)
  Tire_speed_FL/1(Omega_FL) -> Omega_FL/1
  Tb_FR/1 -> Tire_speed_FR/1(Tb_FR)
  Td_FR/1 -> Tire_speed_FR/2(Td_FR)
  Fx_FR/1 -> Tire_speed_FR/3(Fx_FR)
  Tire_speed_FR/1(Omega_FR) -> Omega_FR/1
  Tb_RL/1 -> Tire_speed_RL/1(Tb_RL)
  Fx_RL/1 -> Tire_speed_RL/3(Fx_RL)
  Tire_speed_RL/1(Omega_RL) -> Omega_RL/1
  Tb_RR/1 -> Tire_speed_RR/1(Tb_RR)
  Fx_RR/1 -> Tire_speed_RR/3(Fx_RR)
  Tire_speed_RR/1(Omega_RR) -> Omega_RR/1
  Td_RL/1 -> Tire_speed_RL/2(Td_RL)
  Td_RR/1 -> Tire_speed_RR/2(Td_RR)

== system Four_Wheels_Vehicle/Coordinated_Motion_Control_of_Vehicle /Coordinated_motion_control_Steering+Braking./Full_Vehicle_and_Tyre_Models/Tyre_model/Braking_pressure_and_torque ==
  Mzc_all : Inport
  SteeringAng : Inport  Port=2
  Braking_pressure_and_torque_FL : MATLAB Function  TreatAsAtomicUnit=on
  Braking_pressure_and_torque_FR : MATLAB Function  TreatAsAtomicUnit=on
  Braking_pressure_and_torque_RL : MATLAB Function  TreatAsAtomicUnit=on
  Braking_pressure_and_torque_RR : MATLAB Function  TreatAsAtomicUnit=on
  Demux : Demux
  reff{,1..3} (4 alike) : Constant  Value=reff
  tw{,1..3} (4 alike) : Constant  Value=1.65
  Tb_FL : Outport
  Tb_FR : Outport  Port=2
  Tb_RL : Outport  Port=3
  Tb_RR : Outport  Port=4
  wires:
  Braking_pressure_and_torque_FR/2(Tb_FR) -> Tb_FR/1
  reff1/1 -> Braking_pressure_and_torque_FR/2(reff)
  reff3/1 -> Braking_pressure_and_torque_RR/2(reff)
  tw2/1 -> Braking_pressure_and_torque_RL/3(tw)
  Braking_pressure_and_torque_RR/2(Tb_RR) -> Tb_RR/1
  reff/1 -> Braking_pressure_and_torque_FL/2(reff)
  Braking_pressure_and_torque_FL/2(Tb_FL) -> Tb_FL/1
  tw3/1 -> Braking_pressure_and_torque_RR/3(tw)
  tw1/1 -> Braking_pressure_and_torque_FR/3(tw)
  reff2/1 -> Braking_pressure_and_torque_RL/2(reff)
  Braking_pressure_and_torque_RL/2(Tb_RL) -> Tb_RL/1
  tw/1 -> Braking_pressure_and_torque_FL/3(tw)
  SteeringAng/1 -> Braking_pressure_and_torque_FR/4(SteeringAng), Braking_pressure_and_torque_FL/4(SteeringAng)
  Mzc_all/1 -> Demux/1
  Demux/1 -> Braking_pressure_and_torque_FL/1(M)
  Demux/2 -> Braking_pressure_and_torque_FR/1(M)
  Demux/3 -> Braking_pressure_and_torque_RL/1(M)
  Demux/4 -> Braking_pressure_and_torque_RR/1(M)

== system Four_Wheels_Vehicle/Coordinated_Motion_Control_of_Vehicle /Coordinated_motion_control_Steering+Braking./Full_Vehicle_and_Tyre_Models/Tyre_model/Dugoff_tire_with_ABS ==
  note: Dugoff_Tire_model
  In1 : Inport
  In2 : Inport  Port=2
  In5 : Inport  Port=3
  In3 : Inport  Port=4
  Demux{1..4} (4 alike) : Demux  Outputs=3
  Dugoff_Tire_FL : MATLAB Function  TreatAsAtomicUnit=on
  Dugoff_Tire_FR : MATLAB Function  TreatAsAtomicUnit=on
  Dugoff_Tire_RL : MATLAB Function  TreatAsAtomicUnit=on
  Dugoff_Tire_RR : MATLAB Function  TreatAsAtomicUnit=on
  miu{,1..3} (4 alike) : Constant  Value=miu
  Fx_FL : Outport
  Fx_FR : Outport  Port=2
  Fy_FL : Outport  Port=3
  Fy_FR : Outport  Port=4
  Fx_RL : Outport  Port=5
  Fx_RR : Outport  Port=6
  Fy_RL : Outport  Port=7
  Fy_RR : Outport  Port=8
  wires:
  Demux1/2 -> Dugoff_Tire_RR/2(Fz_RR)
  Demux2/3 -> Dugoff_Tire_FR/3(alpha_FR)
  Demux2/2 -> Dugoff_Tire_FR/2(Fz_FR)
  Demux2/1 -> Dugoff_Tire_FR/1(Sigma)
  Demux3/2 -> Dugoff_Tire_RL/2(Fz_RL)
  Demux4/3 -> Dugoff_Tire_FL/3(alpha_FL)
  Demux4/2 -> Dugoff_Tire_FL/2(Fz_FL)
  Demux4/1 -> Dugoff_Tire_FL/1(Sigma)
  miu1/1 -> Dugoff_Tire_FL/4(miu)
  miu/1 -> Dugoff_Tire_FR/4(miu)
  miu2/1 -> Dugoff_Tire_RL/4(miu)
  miu3/1 -> Dugoff_Tire_RR/4(miu)
  In1/1 -> Demux4/1
  Dugoff_Tire_FL/1(Fx_FL) -> Fx_FL/1
  Dugoff_Tire_FR/1(Fx_FR) -> Fx_FR/1
  Dugoff_Tire_FL/2(Fy_FL) -> Fy_FL/1
  Dugoff_Tire_FR/2(Fy_FR) -> Fy_FR/1
  In5/1 -> Demux1/1
  Dugoff_Tire_RL/1(Fx_RL) -> Fx_RL/1
  Dugoff_Tire_RR/1(Fx_RR) -> Fx_RR/1
  Dugoff_Tire_RL/2(Fy_RL) -> Fy_RL/1
  Dugoff_Tire_RR/2(Fy_RR) -> Fy_RR/1
  In2/1 -> Demux2/1
  Demux3/3 -> Dugoff_Tire_RL/3(alpha_RL)
  Demux3/1 -> Dugoff_Tire_RL/1(Sigma)
  Demux1/1 -> Dugoff_Tire_RR/1(Sigma)
  Demux1/3 -> Dugoff_Tire_RR/3(alpha_RR)
  In3/1 -> Demux3/1

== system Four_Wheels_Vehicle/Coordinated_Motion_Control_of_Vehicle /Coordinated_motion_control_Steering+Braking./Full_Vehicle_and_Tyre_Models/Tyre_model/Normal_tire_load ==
  x_Vel : Inport
  mass : Inport  Port=2
  g : Inport  Port=3
  H_CoG : Inport  Port=4
  beta : Inport  Port=5
  Lf : Inport  Port=6
  Lr : Inport  Port=7
  Hearo : Inport  Port=8
  AirDragConst : Constant  Value=0.3
  Airdensity : Constant  Value=1.22
  Constant : Constant  Value=2
  Constant1 : Constant  Value=2
  Divide : Product  Inputs=*/
  Divide1 : Product  Inputs=*/
  Faero : Subsystem
  FrontalArea : Constant  Value=2
  Fzf : Subsystem
  Fzr : Subsystem
  Scope : Scope
  windVelocity : Constant
  Fz_f : Outport
  Fz_r : Outport  Port=2
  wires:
  Lr/1 -> Fzf/7(Lr), Fzr/9(Lr)
  beta/1 -> Fzf/5(beta), Fzr/7(beta)
  Lf/1 -> Fzf/6(Lf), Fzr/8(Lf)
  Fzf/1(Fz_f) -> Divide/1
  Fzr/1(Fzr) -> Divide1/1
  Constant/1 -> Divide/2
  Constant1/1 -> Divide1/2
  Divide/1 -> Fz_f/1
  Divide1/1 -> Fz_r/1
  g/1 -> Fzf/3(g), Fzr/5(g)
  H_CoG/1 -> Fzf/4(H_CoG), Fzr/6(HatCG)
  Hearo/1 -> Fzf/8(Haero), Fzr/2(Haero)
  mass/1 -> Fzf/2(mass), Fzr/4(mass)
  AirDragConst/1 -> Faero/2(AirDragConst1)
  FrontalArea/1 -> Faero/3(FrontalArea1)
  Airdensity/1 -> Faero/4(Airdensity)
  windVelocity/1 -> Faero/5(windVelocity)
  x_Vel/1 -> Faero/1(Vx), Fzf/1(x_Vel), Fzr/3(xVel)
  Faero/1(Faero) -> Fzr/1(Faero), Fzf/9(Faero), Scope/1

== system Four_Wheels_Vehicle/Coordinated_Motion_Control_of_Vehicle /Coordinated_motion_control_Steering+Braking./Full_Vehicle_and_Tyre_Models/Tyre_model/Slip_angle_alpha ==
  note: Slip_angle_alpha
  x_Vel : Inport
  y_Vel : Inport  Port=2
  yaw_rate : Inport  Port=3
  Steering_Ang. : Inport  Port=4
  Lf : Constant  Value=Lf
  Lr : Constant  Value=Lr
  Slip_angle_alpha : MATLAB Function  TreatAsAtomicUnit=on
  alpha_FL : Outport
  alpha_FR : Outport  Port=2
  alpha_RL : Outport  Port=3
  alpha_RR : Outport  Port=4
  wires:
  Slip_angle_alpha/4(alpha_RR) -> alpha_RR/1
  Slip_angle_alpha/3(alpha_RL) -> alpha_RL/1
  Slip_angle_alpha/2(alpha_FR) -> alpha_FR/1
  Slip_angle_alpha/1(alpha_FL) -> alpha_FL/1
  x_Vel/1 -> Slip_angle_alpha/1(x_Vel)
  y_Vel/1 -> Slip_angle_alpha/2(y_Vel)
  yaw_rate/1 -> Slip_angle_alpha/3(yaw_rate)
  Lf/1 -> Slip_angle_alpha/4(Lf)
  Lr/1 -> Slip_angle_alpha/5(Lr)
  Steering_Ang./1 -> Slip_angle_alpha/6(deltaw)

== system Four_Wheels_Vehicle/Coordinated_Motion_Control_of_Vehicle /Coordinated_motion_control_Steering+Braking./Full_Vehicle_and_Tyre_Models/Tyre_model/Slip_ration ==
  note: Slip_ration
  Omega_FL : Inport
  Omega_FR : Inport  Port=2
  Omega_RL : Inport  Port=3
  Omega_RR : Inport  Port=4
  x_Vel : Inport  Port=5
  Slip_ration_Sigma : MATLAB Function  TreatAsAtomicUnit=on
  reff : Constant  Value=reff
  Sigma_FL : Outport
  Sigma_FR : Outport  Port=2
  Sigma_RL : Outport  Port=3
  Sigma_RR : Outport  Port=4
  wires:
  reff/1 -> Slip_ration_Sigma/6(reff)
  Slip_ration_Sigma/2(Sigma_FR) -> Sigma_FR/1
  Slip_ration_Sigma/3(Sigma_RL) -> Sigma_RL/1
  Slip_ration_Sigma/4(Sigma_RR) -> Sigma_RR/1
  Slip_ration_Sigma/1(Sigma_FL) -> Sigma_FL/1
  Omega_FL/1 -> Slip_ration_Sigma/1(Omega_FL)
  Omega_RL/1 -> Slip_ration_Sigma/3(Omega_RL)
  Omega_RR/1 -> Slip_ration_Sigma/4(Omega_RR)
  Omega_FR/1 -> Slip_ration_Sigma/2(Omega_FR)
  x_Vel/1 -> Slip_ration_Sigma/5(x_Vel)

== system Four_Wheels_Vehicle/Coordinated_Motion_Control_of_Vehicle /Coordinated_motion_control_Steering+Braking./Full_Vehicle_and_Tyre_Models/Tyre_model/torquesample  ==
  Demux : Demux  Tag=STV Demux  Outputs=1
  FromWs : FromWorkspace  Tag=STV FromWs  VariableName=tuvar  SampleTime=0  SigBuilderData=DataTag16  VnvData=DataTag17
  Signal 1 : Outport  Tag=STV Outport
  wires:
  FromWs/1 -> Demux/1
  Demux/1 -> Signal 1/1

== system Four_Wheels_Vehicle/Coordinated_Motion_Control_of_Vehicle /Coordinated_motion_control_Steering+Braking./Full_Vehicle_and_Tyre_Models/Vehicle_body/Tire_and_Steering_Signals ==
  Steering_Ang. : Inport
  Fx_and_Fy : Inport  Port=2
  Demux : Demux  Outputs=8
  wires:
  Steering_Ang./1 -> [SteeringAng]
  Demux/1 -> [Fx_FL]
  Demux/2 -> [Fx_FR]
  Demux/3 -> [Fy_FL]
  Demux/4 -> [Fy_FR]
  Demux/5 -> [Fx_RL]
  Demux/6 -> [Fx_RR]
  Demux/7 -> [Fy_RL]
  Demux/8 -> [Fy_RR]
  Fx_and_Fy/1 -> Demux/1

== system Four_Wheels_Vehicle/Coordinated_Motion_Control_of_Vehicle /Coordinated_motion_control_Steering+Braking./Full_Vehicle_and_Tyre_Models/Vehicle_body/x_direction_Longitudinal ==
  note: x_direction_Longitudinal
  Fx_FL : Inport
  Fx_FR : Inport  Port=2
  Fy_FL : Inport  Port=3
  Fy_FR : Inport  Port=4
  Fx_RL : Inport  Port=5
  Fx_RR : Inport  Port=6
  Steering_Ang. : Inport  Port=7
  yaw_rate : Inport  Port=8
  y_Vel : Inport  Port=9
  1/m : Gain  Gain=1/1750
  Add : Sum
  Add1 : Sum
  Add2 : Sum  Inputs=+-++
  Add3 : Sum
  Product : Product
  Product1 : Product
  Product18 : Product
  Stop Simulation : Stop
  Vx0 : Integrator  InitialCondition=5  UpperSaturationLimit=100  LowerSaturationLimit=0  ShowSaturationPort=on
  cos_deltaw : Fcn  Expr=cos(u)
  sin_deltaw : Fcn  Expr=sin(u)
  x_Vel : Outport
  x total force : Outport  Port=2
  dx : Outport  Port=3
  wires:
  Product18/1 -> Add3/2
  Vx0/1 -> x_Vel/1
  Vx0/2 -> Stop Simulation/1
  Add3/1 -> dx/1, Vx0/1
  1/m/1 -> Add3/1
  Add2/1 -> 1/m/1, x total force/1
  cos_deltaw/1 -> Product/2
  Add/1 -> Product/1
  Steering_Ang./1 -> cos_deltaw/1, sin_deltaw/1
  yaw_rate/1 -> Product18/1
  y_Vel/1 -> Product18/2
  Add1/1 -> Product1/1
  sin_deltaw/1 -> Product1/2
  Fy_FL/1 -> Add1/1
  Fy_FR/1 -> Add1/2
  Fx_FL/1 -> Add/1
  Fx_FR/1 -> Add/2
  Product/1 -> Add2/1
  Product1/1 -> Add2/2
  Fx_RL/1 -> Add2/3
  Fx_RR/1 -> Add2/4
